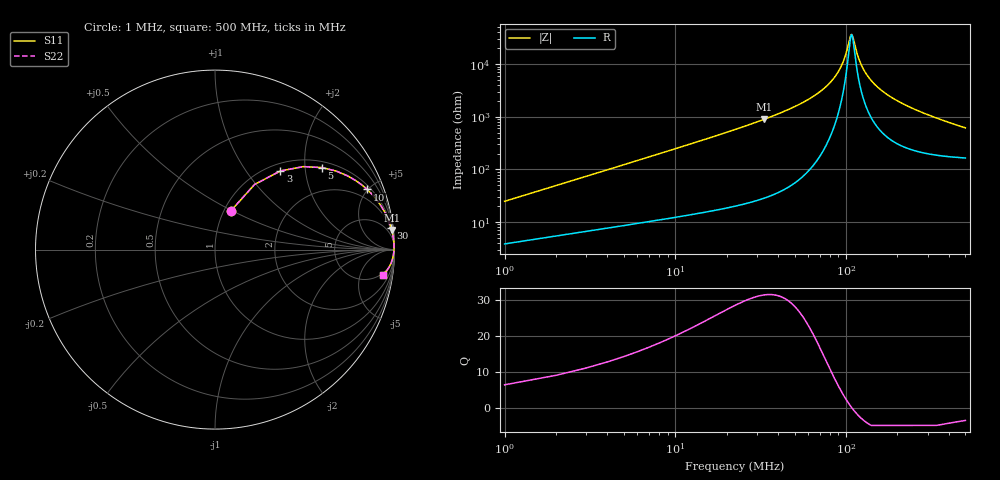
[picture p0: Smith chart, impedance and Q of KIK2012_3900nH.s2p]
!version-2
!date-01.2022
!Series
# MHz S RI R 50
!Freq ReS11 ImS11 ReS21 ImS21 ReS12 ImS12 ReS22 ImS22
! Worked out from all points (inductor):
!   500 points, 1 MHz to 500 MHz, reference 50 ohm
!   read as one part in series: L = 3.9 uH near 3 MHz
!   highest Q = 31.5 at 33 MHz (marker M1), where L = 4.3 uH
!   self-resonance near 107 MHz
!   S11 on the Smith chart (normalised r, x): 1 MHz: 1.08, +0.49; 3 MHz: 1.13, +1.47; 5 MHz: 1.17, +2.46; 10 MHz: 1.25, +4.94; 30 MHz: 2, +16; 500 MHz: 4, -12
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1  0.0878 0.2153  0.9122 -0.2153  0.9122 -0.2153  0.0878 0.2153
3  0.3647 0.4383  0.6353 -0.4383  0.6353 -0.4383  0.3647 0.4383
5  0.5958 0.457  0.4042 -0.457  0.4042 -0.457  0.5958 0.457
7  0.7365 0.4119  0.2635 -0.4119  0.2635 -0.4119  0.7365 0.4119
10  0.8476 0.3354  0.1524 -0.3354  0.1524 -0.3354  0.8476 0.3354
17  0.9405 0.2178  0.0595 -0.2178  0.0595 -0.2178  0.9405 0.2178
30  0.9807 0.1225  0.0193 -0.1225  0.0193 -0.1225  0.9807 0.1225
33  0.9842 0.1098  0.0158 -0.1098  0.0158 -0.1098  0.9842 0.1098
70  0.9969 0.0335  0.00311 -0.0335  0.00311 -0.0335  0.9969 0.0335
85  0.9975 0.0181  0.00247 -0.0181  0.00247 -0.0181  0.9975 0.0181
95  0.9976 0.00956  0.00244 -0.00956  0.00244 -0.00956  0.9976 0.00956
105  0.9974 0.00201  0.00263 -0.00201  0.00263 -0.00201  0.9974 0.00201
108  0.9973 -9.95e-05  0.00272 9.95e-05  0.00272 9.95e-05  0.9973 -9.95e-05
119  0.9968 -0.00737  0.00315 0.00737  0.00315 0.00737  0.9968 -0.00737
129  0.9963 -0.0135  0.00368 0.0135  0.00368 0.0135  0.9963 -0.0135
145  0.9953 -0.0224  0.00473 0.0224  0.00473 0.0224  0.9953 -0.0224
168  0.9934 -0.0339  0.00662 0.0339  0.00662 0.0339  0.9934 -0.0339
203  0.9898 -0.0496  0.0102 0.0496  0.0102 0.0496  0.9898 -0.0496
251  0.9837 -0.0686  0.0163 0.0686  0.0163 0.0686  0.9837 -0.0686
334  0.9705 -0.0968  0.0295 0.0968  0.0295 0.0968  0.9705 -0.0968
417  0.9548 -0.1206  0.0452 0.1206  0.0452 0.1206  0.9548 -0.1206
500  0.9373 -0.1404  0.0627 0.1404  0.0627 0.1404  0.9373 -0.1404
